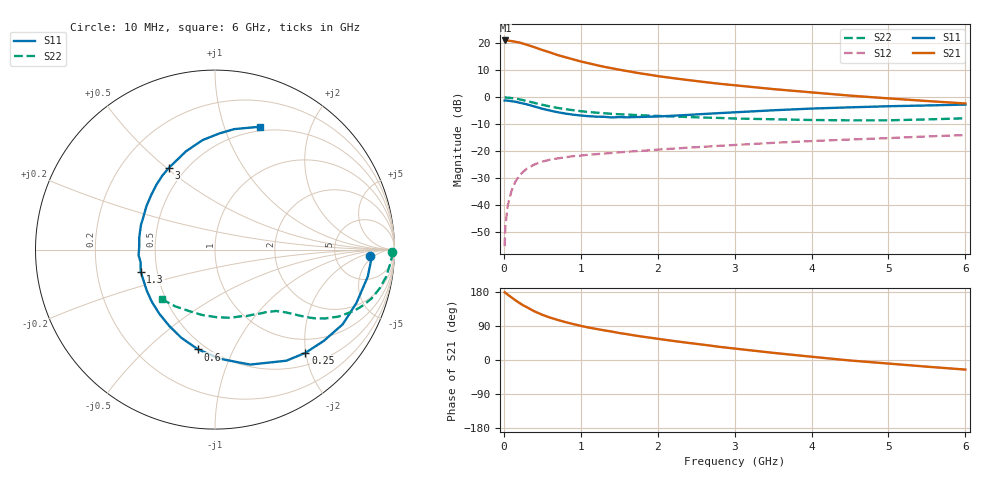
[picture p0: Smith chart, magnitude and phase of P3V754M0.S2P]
! SIEMENS Small Signal Semiconductors
! BFP181
! Si NPN RF Bipolar Junction Transistor in SOT143
! VCE = 0.75 V  IC = 4 mA
! Common Emitter S-Parameters:  March  1996
# GHz  S  MA  R  50
!  f  S11  S21  S12  S22
! GHz  MAG  ANG  MAG  ANG  MAG  ANG  MAG  ANG
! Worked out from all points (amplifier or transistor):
!   36 points, 10 MHz to 6 GHz, reference 50 ohm
!   highest |S21| = 21.1 dB at 20 MHz (marker M1)
!   |S21| within 3 dB of that: start of sweep to 446 MHz
!   unconditionally stable (mu >= 1): 1.469 GHz to end of sweep
!   at 250 MHz: K = 0.23, MSG = 23.9 dB, |S12| = -27.8 dB
!   at 1.4 GHz: K = 0.98, MSG = 15.8 dB, |S12| = -20.7 dB
!   at 6 GHz: K = 1.19, MAG = 3.3 dB, |S12| = -14.1 dB
!   S11 on the Smith chart (normalised r, x): 10 MHz: 13, -3; 250 MHz: 0.72, -1.99; 600 MHz: 0.45, -0.74; 1.3 GHz: 0.40, -0.12; 3 GHz: 0.41, +0.51; 6 GHz: 0.45, +1.33
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0.01  0.8653 -2.2  11.34 178.7  0.0017 85.3  0.9843 -0.8
0.02  0.8711 -4.3  11.34 177.5  0.004 84.1  0.988 -1.9
0.05  0.8644 -10.0  11.29 172.5  0.0096 84.2  0.9794 -4.6
0.1  0.8424 -20.6  11.03 165.1  0.0183 78.6  0.965 -9.1
0.15  0.8244 -30.3  10.72 157.7  0.0267 72.3  0.943 -13.2
0.2  0.7912 -40.0  10.42 150.9  0.0348 69.0  0.915 -17.2
0.25  0.7646 -48.8  9.898 144.4  0.0407 63.6  0.8812 -20.7
0.4  0.6699 -73.0  8.477 128.1  0.0563 53.2  0.7825 -28.5
0.5  0.6095 -87.2  7.537 119.3  0.0634 47.8  0.7223 -32.1
0.6  0.5642 -99.6  6.797 112.0  0.0689 44.4  0.672 -34.7
0.7  0.526 -110.9  6.063 105.7  0.0728 41.3  0.6316 -36.5
0.8  0.4956 -121.0  5.539 100.0  0.0765 38.9  0.5996 -37.9
0.9  0.4734 -130.9  5.055 94.9  0.0801 37.4  0.5732 -39.1
1.1  0.4439 -148.7  4.283 85.7  0.0851 35.1  0.5311 -41.3
1.3  0.432 -163.3  3.682 78.4  0.0894 33.1  0.5036 -43.4
1.7  0.4273 171.2  2.892 64.8  0.099 31.6  0.4672 -47.6
2.2  0.4522 147.7  2.26 50.4  0.1106 29.9  0.4378 -54.2
3  0.5233 119.3  1.667 30.2  0.1293 26.5  0.4014 -67.3
3.5  0.5708 106.5  1.415 18.9  0.1417 24.3  0.3889 -77.6
4.5  0.6474 87.9  1.07 -1.3  0.1634 18.1  0.3713 -101.2
5.5  0.7018 75.1  0.849 -17.6  0.1864 12.7  0.3862 -125.2
6  0.7289 69.9  0.764 -25.3  0.1978 9.1  0.4054 -137.0
